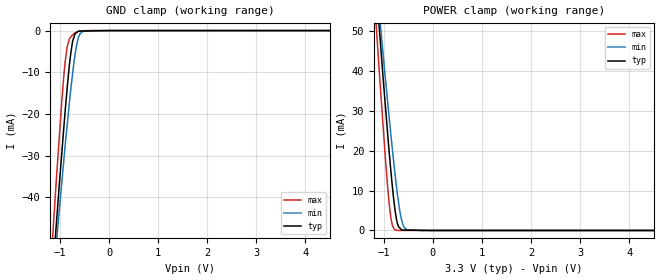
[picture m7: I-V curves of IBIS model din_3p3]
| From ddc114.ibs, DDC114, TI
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|   din_3p3 Model
[Model]   din_3p3
Model_type   Input
Vinl = 0.66
Vinh = 2.64
|   typ   min   max
|   (nom PVT)   (fast PVT)   (slow PVT)
|C_comp from frequency sweep method (F=55.6MHz)
|Average
|C_comp   1.657e-12   1.558e-12   1.758e-12
|C_comp from LC tank measurement(L=1nH)
|Average
|Resonant Frequency(Hz)   9.160e+09   9.220e+09   8.910e+09
C_comp   3.022e-13   2.983e-13   3.194e-13
| Where nom  PVT is Nominal Process, 3.3V, 27C
|   Fast PVT is Strong Process,  3.6V, -40C
|   Slow PVT is Weak Process,   3V, 87C
[Model Spec]
|Subparameter   typ   min   max
Vinl   0.66   0.60   0.72
Vinh   2.64   2.4   2.88
[Voltage Range]   3.3   3   3.6
|Ambient Temperature   25   85   -40
|Junction Temperature
[Temperature Range]   27   87   -40
[Power Clamp Reference]   3.3   3   3.6
[GND Clamp Reference]   0   0   0
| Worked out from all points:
|   GND clamp passes 1 mA (typ) near -0.70 V on its own axis
|   POWER clamp passes 1 mA (typ) near -0.70 V on its own axis
[GND Clamp]
|   Voltage   I(typ)   I(min)   I(max)
-3.3V     -422.8mA   -361.6mA   -470.1mA
-1.145V   -57.41mA   -59.88mA   -48.25mA
-1.069V   -45.3mA    -50mA      -34.51mA
-1.003V   -35.01mA   -41.41mA   -23.34mA
-928.8mV  -24.01mA   -31.73mA   -11.56mA
-856.8mV  -13.9mA    -22.79mA   -3.938mA
-745.8mV  -2.663mA   -10.37mA   -1.071mA
-684mV    -675.1uA   -4.868mA   -455.4uA
-627mV    -128.4uA   -1.704mA   -228.8uA
-537mV    -109.9uA   -201.5uA   -37.41uA
-285mV    -58.01uA   -143.3nA   -354.6nA
6.6V      0A         0A         0A
[POWER Clamp]
|   Voltage   I(typ)   I(min)   I(max)
-3.3V     428.6mA    367.2mA    475.9mA
-1.152V   60.24mA    62.56mA    50.85mA
-1.084V   49.33mA    53.37mA    38.23mA
-1.006V   36.99mA    43.17mA    24.7mA
-896.4mV  20.41mA    28.93mA    7.343mA
-828mV    11.26mA    20.54mA    1.333mA
-774mV    5.272mA    14.33mA    200.9uA
-726mV    1.869mA    9.333mA    30.3uA
-648mV    317.1uA    3.13mA     1.196uA
-591mV    105.3uA    920.5uA    247.9nA
-531mV    94.51uA    206.3uA    150.1nA
6.6V      0A         0A         0A
